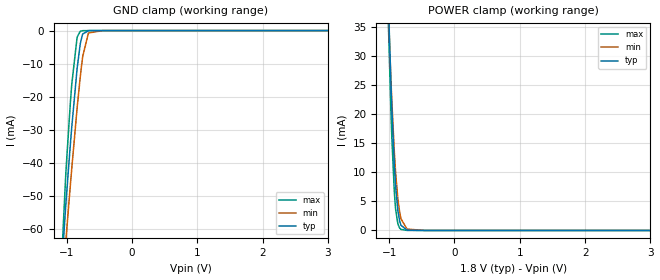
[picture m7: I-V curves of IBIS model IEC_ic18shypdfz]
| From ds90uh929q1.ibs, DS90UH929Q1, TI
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|   Model
[Model]   IEC_ic18shypdfz
Model_type   Input
Vinl = 0.54
Vinh = 1.26
|   typ   min   max
C_comp   0.246pF   0.216pF   0.318pF
[Voltage Range]   1.8   1.71   1.89
[Temperature Range]   27   105   -40
[Power Clamp Reference]   1.8   1.71   1.89
[GND Clamp Reference]   0   0   0
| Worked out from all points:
|   GND clamp passes 1 mA (typ) near -0.75 V on its own axis
|   POWER clamp passes 1 mA (typ) near -0.82 V on its own axis
[GND Clamp]
|   Voltage   I(typ)   I(min)   I(max)
-1.8V     -460.2mA   -412.9mA   -493.3mA
-1.076V   -72.12mA   -80.05mA   -69.52mA
-1.017V   -54.01mA   -64.86mA   -45.16mA
-1.006V   -51mA      -62.17mA   -41.29mA
-941.4mV  -34.14mA   -46.46mA   -21.5mA
-919.8mV  -28.91mA   -41.38mA   -16.05mA
-838.8mV  -11.41mA   -23.39mA   -1.974mA
-790.2mV  -3.928mA   -13.88mA   -194.7uA
-752.4mV  -1.035mA   -7.727mA   -30.55uA
-666mV    -20.55uA   -730.7uA   -1.448uA
-444.6mV  -443.3nA   -522.5nA   -544.6nA
3.6V      0A         0A         0A
[POWER Clamp]
|   Voltage   I(typ)   I(min)   I(max)
-1.8V     424.7mA    379.5mA    464.9mA
-1.017V   41.05mA    39.48mA    37.84mA
-973.8mV  25.84mA    26.39mA    21.06mA
-957.6mV  20.86mA    22.06mA    15.8mA
-919.8mV  11.28mA    13.48mA    6.595mA
-898.2mV  7.308mA    9.648mA    3.477mA
-865.8mV  3.396mA    5.426mA    1.141mA
-838.8mV  1.647mA    3.159mA    417.2uA
-817.2mV  891.3uA    1.986mA    183.3uA
-725.4mV  59.21uA    236.8uA    8.171uA
-444.6mV  2.25uA     2.052uA    2.871uA
3.6V      0A         0A         0A
